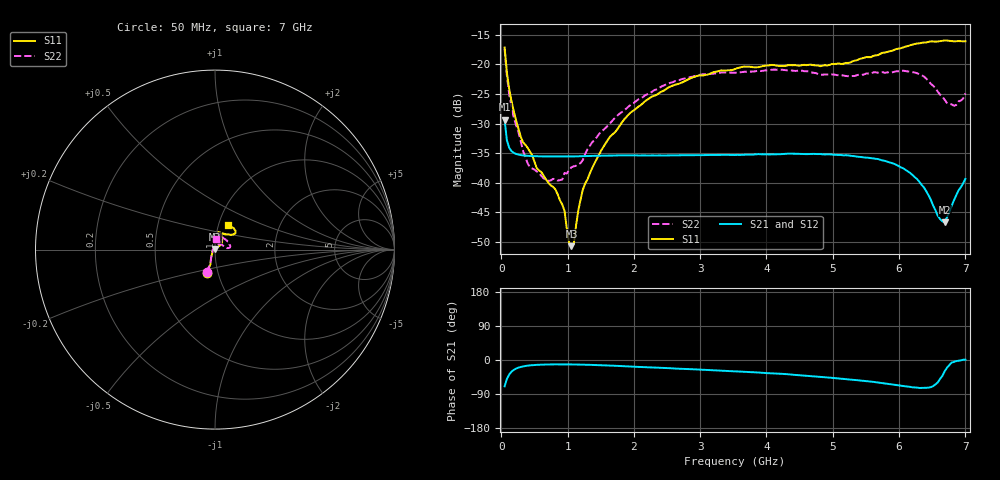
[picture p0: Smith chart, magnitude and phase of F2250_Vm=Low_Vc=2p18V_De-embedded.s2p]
! Integrated Device Technology
! Corporate Headquarters
! 6024 Silver Creek Valley Road
! San Jose, CA 95138  USA
! Phone:  1-408-284-8200
! Toll Free:  1-800-223-1366
! Webpage:  http://www.idt.com/
! Timing and RF Division
! 515 Groton Road, Suite 102
! Westford, MA 01886-6024
! Device:  F2250
! Description: Voltage Variable RF Attenuator
! Frequency:  50.0 -  6000.00 MHz
! Package:  3x3 mm Thin QFN Plastic Package: 16 pin
! Ports:  2 RF, 3 DC
!  Pin  1  = GND
!  Pin  2  = NC
!  Pin  3  = RF1  = Port 1
!  Pin  4  = NC
!  Pin  5  = GND
!  Pin  6  = GND
!  Pin  7  = GND
!  Pin  8  = GND
!  Pin  9  = NC
!  Pin 10  = RF2  = Port 2
!  Pin 11  = NC
!  Pin 12  = GND
!  Pin 13  = GND
!  Pin 14  = VCNTRL
!  Pin 15  = VDD
!  Pin 16  = VMODE
! Vcntrl:  2.180 Volts
! Vmode:  +0.000 Volts
! Vdd:  +3.30  Volts
! Current:  1.178 mA
! Data:  The device was measured on a the F2250 evaluation board which has
!  individual transmission lines to the RF pins.  Data was collected
!  using a calibrated network analyzer.  The evaluation board was
!  de-embedded using a TRL calibration technique.
!  The reference plane is the edge of the package pin.
! Misc:  SN 10
!  Action Tracker AT0258
! Date Measured:  2014-11-26
! Date:  2015-10-15  MJV
! Note:
!  Integrated Device Technology supplies this data as a sample of measured
!  data at the package pin for this product.  Your particular data for this
!  product may vary.
!  Data was taken at 25 degrees C.
!  Integrated Device Technology reserves the right to change this data at anytime.
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# GHz S dB R 50
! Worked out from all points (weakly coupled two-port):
!   201 points, 50 MHz to 7 GHz, reference 50 ohm
!   highest |S21| = -29.37 dB at 50 MHz (marker M1); lowest = -46.6 dB at 6.687 GHz (marker M2)
!   lowest |S11| = -50.7 dB at 1.058 GHz (marker M3), VSWR 1.01, Z = 49.8 + j0.246 ohm
!   |S11| at or under -10 dB: start of sweep to end of sweep
!   |S22| runs from -39.7 to -17.4 dB; largest |S21 - S12| = 7e-05
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0.05  -17.18 -108.6  -29.37 -69.4  -29.37 -69.4  -17.43 -110.3
0.08475  -21.44 -107.4  -32.84 -49.9  -32.84 -49.9  -21.97 -108.5
0.189  -28.00 -119.6  -34.95 -26.0  -34.95 -26.0  -29.01 -122.9
0.29325  -32.21 -127.7  -35.32 -18.3  -35.32 -18.3  -32.99 -131.8
0.3975  -34.09 -141.7  -35.44 -14.9  -35.44 -14.9  -36.71 -155.6
0.71025  -39.97 -168.3  -35.56 -11.8  -35.56 -11.8  -39.66 152.2
0.91875  -43.64 158.1  -35.57 -11.6  -35.57 -11.6  -39.45 123.9
0.9535  -44.70 169.5  -35.57 -11.6  -35.57 -11.6  -38.34 122.4
1.023  -50.08 144.2  -35.56 -11.7  -35.56 -11.6  -37.87 104.9
1.05775  -50.68 122.3  -35.56 -11.7  -35.56 -11.7  -37.37 99.7
1.0925  -50.35 90.1  -35.55 -11.8  -35.54 -11.8  -37.22 94.6
1.162  -44.63 57.0  -35.53 -12.0  -35.53 -12.0  -36.86 83.4
1.2315  -41.10 44.0  -35.50 -12.2  -35.50 -12.2  -36.10 74.3
1.6485  -32.11 41.9  -35.41 -14.8  -35.41 -14.8  -29.87 58.7
2.37825  -24.87 47.3  -35.37 -20.5  -35.38 -20.5  -24.05 53.9
3.525  -20.80 72.5  -35.31 -29.8  -35.30 -29.8  -21.43 73.3
4.7065  -20.17 72.4  -35.12 -42.8  -35.11 -42.8  -21.44 71.5
5.85325  -17.82 40.5  -36.54 -63.5  -36.53 -63.5  -21.32 21.5
6.27025  -16.51 40.1  -39.35 -72.8  -39.35 -72.8  -21.52 8.1
6.68725  -15.99 48.8  -46.64 -29.8  -46.62 -29.5  -25.99 27.2
6.82625  -16.14 53.6  -42.96 -5.0  -42.91 -4.8  -27.00 52.8
7  -16.12 63.3  -39.33 0.6  -39.30 0.5  -24.93 84.2
